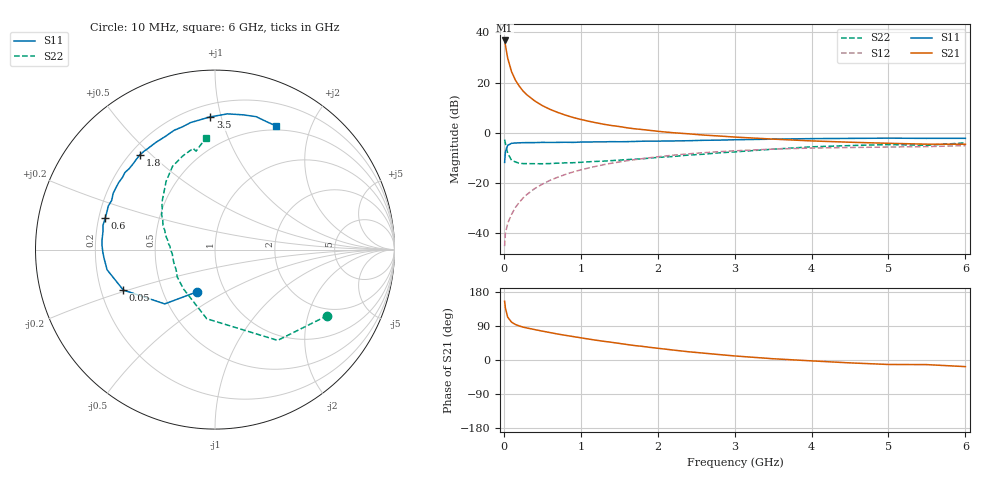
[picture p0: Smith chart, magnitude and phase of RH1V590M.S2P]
! SIEMENS Small Signal Semiconductors
! BFR106
! Si NPN RF Bipolar Junction Transistor in SOT23
! VCE = 1.5 V  IC = 90 mA
! Common Emitter S-Parameters:  August  1996
# GHz  S  MA  R  50
!  f  S11  S21  S12  S22
! GHz  MAG  ANG  MAG  ANG  MAG  ANG  MAG  ANG
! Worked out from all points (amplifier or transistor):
!   36 points, 10 MHz to 6 GHz, reference 50 ohm
!   highest |S21| = 36.8 dB at 10 MHz (marker M1)
!   |S21| within 3 dB of that: start of sweep to 26.81 MHz
!   unconditionally stable (mu >= 1): 111 MHz to end of sweep
!   at 250 MHz: K = 1.13, MAG = 19.2 dB, |S12| = -26.1 dB
!   at 1.4 GHz: K = 1.11, MAG = 5.5 dB, |S12| = -12.2 dB
!   at 6 GHz: K = 1.03, MAG = -0.7 dB, |S12| = -5.2 dB
!   S11 on the Smith chart (normalised r, x): 10 MHz: 0.74, -0.37; 50 MHz: 0.29, -0.19; 600 MHz: 0.23, +0.13; 1.8 GHz: 0.24, +0.46; 3.5 GHz: 0.28, +0.92; 6 GHz: 0.45, +1.51
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0.01  0.2543 -112.7  69.31 155.1  0.0054 69.2  0.7262 -30.4
0.02  0.4121 -132.8  56.29 137.4  0.0097 62.0  0.6146 -55.4
0.05  0.5584 -156.2  30.73 113.1  0.0154 57.2  0.3879 -96.8
0.1  0.6117 -169.4  16.54 99.8  0.0232 64.2  0.2809 -128.6
0.15  0.6209 -176.0  11.22 93.7  0.032 68.2  0.26 -144.1
0.2  0.6258 -179.1  8.49 89.9  0.0404 70.5  0.2441 -152.4
0.25  0.6299 177.7  6.782 86.7  0.0495 71.2  0.2409 -159.4
0.3  0.6318 175.6  5.691 84.5  0.0582 72.4  0.2406 -162.8
0.4  0.632 171.1  4.311 80.3  0.0761 72.9  0.2395 -169.1
0.5  0.6385 167.8  3.469 76.2  0.0935 72.0  0.2391 -173.4
0.6  0.6366 164.1  2.916 72.4  0.1115 71.0  0.2412 -176.1
0.7  0.638 160.5  2.534 68.5  0.1285 69.7  0.2456 -178.5
0.8  0.6423 157.9  2.238 65.1  0.1462 68.0  0.2492 178.5
1.1  0.6508 148.0  1.691 55.3  0.1967 63.1  0.2615 172.7
1.4  0.6607 139.5  1.386 46.7  0.2446 57.5  0.276 166.7
1.8  0.6736 128.4  1.152 36.0  0.3023 50.2  0.3005 158.8
2.2  0.6824 118.6  0.996 26.3  0.3545 42.9  0.3337 150.7
2.8  0.7078 104.8  0.856 14.3  0.4164 32.3  0.3951 138.5
3.5  0.7402 92.0  0.742 3.3  0.4691 21.0  0.4673 125.7
4.5  0.767 78.2  0.643 -7.6  0.5043 7.0  0.5516 109.1
5.5  0.7681 67.6  0.588 -12.2  0.5256 -1.2  0.5584 100.9
6  0.7688 63.9  0.586 -17.5  0.5493 -7.7  0.6252 94.6
